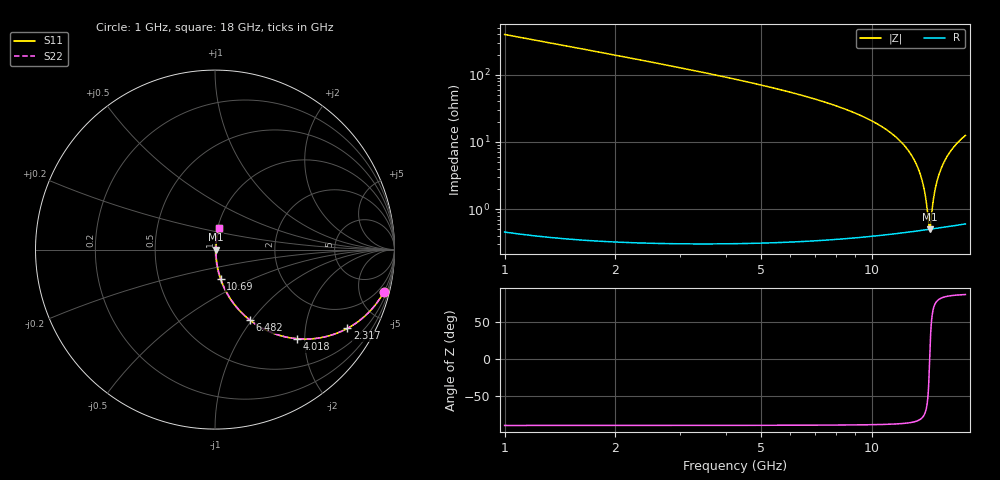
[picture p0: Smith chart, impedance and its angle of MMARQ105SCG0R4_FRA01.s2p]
! MMARQ105SCG0R4_FRA01  S-PARAMETER MODEL  ( Standard Model )
! Model Generated by TAIYO YUDEN Corporation (http://www.ty-top.com)
! Version 1.0
! TAIYO YUDEN Control No. 230906
! Copyright(c) 2023 TAIYO YUDEN CO.,LTD. All Rights Reserved.
! Product Description (link to TY-COMPAS)
! https://ds.yuden.co.jp/TYCOMPAS/or/detail?pn=MMARQ105SCG0R4BFRA01&u=M
! Products Name : Multilayer Ceramic Capacitors
! Characteristics :
!  Capacitance : 0.4 [pF] , Rated Voltage : 250 [V] , TCC : CG / C0G
!  Case Size : 1.0 x 0.5 / 0.039 x 0.02 [mm/inch] , Thickness : 0.5 / 0.02 [mm/inch]
!  (Conditions: Temperature = 25 [degC] , DC Bias Voltage = 0 [V])
! External Node Assignments :
!  1  o---| |---o  2
! GND o---------o GND
! Frequency Range : 1000MHz  -  18000MHz  [ 401 STEP ]
# MHZ S RI R 50
! Freq[MHz].  S11 Real  S11 Imag  S21 Real  S21 Imag  S12 Real  S12 Imag  S22 Real  S22 Imag
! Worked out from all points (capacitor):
!   401 points, 1 GHz to 18 GHz, reference 50 ohm
!   read as one part in series: C = 398 fF near 1.085 GHz
!   lowest |Z| = 502 mohm at 14.39 GHz (marker M1)
!   series resonance near 14.39 GHz, so ESL is about 310 pH
!   S11 on the Smith chart (normalised r, x): 1 GHz: 1.01, -7.95; 2.317 GHz: 1.01, -3.36; 4.018 GHz: 1.01, -1.83; 6.482 GHz: 1.01, -0.98; 10.69 GHz: 1.01, -0.33; 18 GHz: 1.01, +0.25
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1000  0.9403 -0.2364  0.0597 0.2364  0.0597 0.2364  0.9403 -0.2364
1595  0.8592 -0.3471  0.1408 0.3471  0.1408 0.3471  0.8592 -0.3471
2317.5  0.7378 -0.4389  0.2622 0.4389  0.2622 0.4389  0.7378 -0.4389
3847.5  0.4817 -0.4981  0.5183 0.4981  0.5183 0.4981  0.4817 -0.4981
4017.5  0.4567 -0.4965  0.5433 0.4965  0.5433 0.4965  0.4567 -0.4965
6482.5  0.1958 -0.3935  0.8042 0.3935  0.8042 0.3935  0.1958 -0.3935
6695  0.1809 -0.3814  0.8191 0.3814  0.8191 0.3814  0.1809 -0.3814
9500  0.0564 -0.2227  0.9436 0.2227  0.9436 0.2227  0.0564 -0.2227
10690  0.0309 -0.1613  0.9691 0.1613  0.9691 0.1613  0.0309 -0.1613
12347.5  0.0116 -0.0837  0.9884 0.0837  0.9884 0.0837  0.0116 -0.0837
13070  0.00744 -0.0526  0.9926 0.0526  0.9926 0.0526  0.00744 -0.0526
13622.5  0.00569 -0.03  0.9943 0.03  0.9943 0.03  0.00569 -0.03
13962.5  0.00515 -0.0164  0.9948 0.0164  0.9948 0.0164  0.00515 -0.0164
14302.5  0.00498 -0.00324  0.995 0.00324  0.995 0.00324  0.00498 -0.00324
14387.5  0.00499 5.55e-06  0.995 -5.55e-06  0.995 -5.55e-06  0.00499 5.55e-06
14472.5  0.00502 0.00323  0.995 -0.00323  0.995 -0.00323  0.00502 0.00323
14685  0.0052 0.0112  0.9948 -0.0112  0.9948 -0.0112  0.0052 0.0112
14812.5  0.00536 0.016  0.9946 -0.016  0.9946 -0.016  0.00536 0.016
15195  0.00611 0.0299  0.9939 -0.0299  0.9939 -0.0299  0.00611 0.0299
15662.5  0.00751 0.0465  0.9925 -0.0465  0.9925 -0.0465  0.00751 0.0465
16257.5  0.01 0.0667  0.99 -0.0667  0.99 -0.0667  0.01 0.0667
18000  0.0211 0.1216  0.9789 -0.1216  0.9789 -0.1216  0.0211 0.1216
